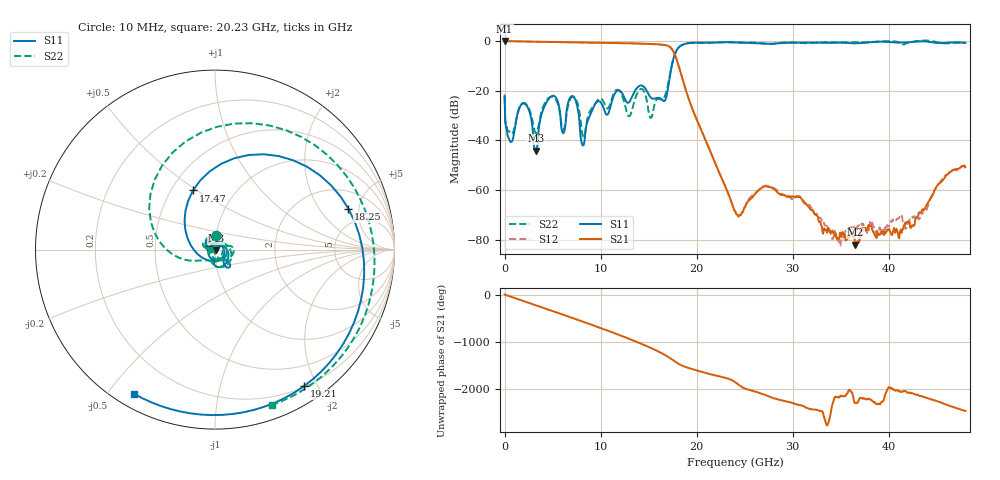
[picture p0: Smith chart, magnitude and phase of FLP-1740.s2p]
! MARKI MICROWAVE INC.
! Email:  info@markimicrowave.com  Phone:  408-778-4200
! Model Number:  FLP-1740  Date:  05/11
! Filename:		FLP-1740.S2P  Version: 1.0
! Description:  2-port S-parameter data for Low Pass Filter FLP-1740
! Features:		Low Insertion Loss, High Stop Band Rejection, Excellent Return Loss, 15th Order Filter
! Frequency Range: 	10 MHz to 48 GHz
! Measurements:		S11, S21, S12, S22
# Hz S  dB  R 50
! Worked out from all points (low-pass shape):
!   801 points, 10 MHz to 48 GHz, reference 50 ohm
!   highest |S21| = 0.00 dB at 10 MHz (marker M1); lowest = -82.1 dB at 36.54 GHz (marker M2)
!   |S21| within 3 dB of the highest: start of sweep to 17.38 GHz
!   lowest |S11| = -44.2 dB at 3.249 GHz (marker M3), VSWR 1.01, Z = 50.5 - j0.309 ohm
!   |S11| at or under -10 dB: start of sweep to 17.42 GHz
!   |S22| runs from -38.5 to 0.2 dB; largest |S21 - S12| = 0.0033
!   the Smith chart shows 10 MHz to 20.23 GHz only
!   S11 on the Smith chart (normalised r, x): 10 MHz: 1.00, +0.16; 17.47 GHz: 0.64, +0.48; 18.25 GHz: 3.36, +3.87; 19.21 GHz: 0.21, -1.83; 20.23 GHz: 0.05, -0.58
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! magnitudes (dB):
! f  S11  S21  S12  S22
! 10 MHz  -22.0  0.0  0.0  -22.2
! 669.9 MHz  -40.7  -0.1  -0.1  -37.3
! 2.23 GHz  -25.7  -0.2  -0.2  -25.3
! 3.249 GHz  -44.2  -0.3  -0.3  -37.1
! 4.989 GHz  -22.1  -0.4  -0.4  -22.5
! 6.129 GHz  -37.1  -0.5  -0.5  -35.7
! 7.268 GHz  -22.9  -0.5  -0.6  -22.6
! 8.048 GHz  -41.3  -0.6  -0.6  -36.3
! 11.77 GHz  -20.0  -0.8  -0.9  -19.6
! 12.97 GHz  -24.7  -0.9  -0.9  -30.4
! 14.11 GHz  -18.0  -1.1  -1.1  -19.5
! 16.03 GHz  -22.9  -1.4  -1.4  -23.3
! 17.47 GHz  -9.1  -3.4  -3.4  -9.1
! 18.25 GHz  -2.2  -11.5  -11.5  -2.2
! 19.21 GHz  -0.8  -23.5  -23.5  -0.9
! 20.23 GHz  -0.7  -33.5  -33.5  -0.7
! 24 GHz  -0.6  -68.6  -68.5  -0.5
! 27.18 GHz  -1.1  -58.5  -58.2  -1.1
! 32.04 GHz  -0.7  -68.1  -68.0  -0.7
! 36.54 GHz  -0.9  -82.1  -74.5  -0.5
! 40.02 GHz  -0.4  -75.7  -74.5  0.0
! 48 GHz  -0.7  -50.7  -51.3  -0.7
